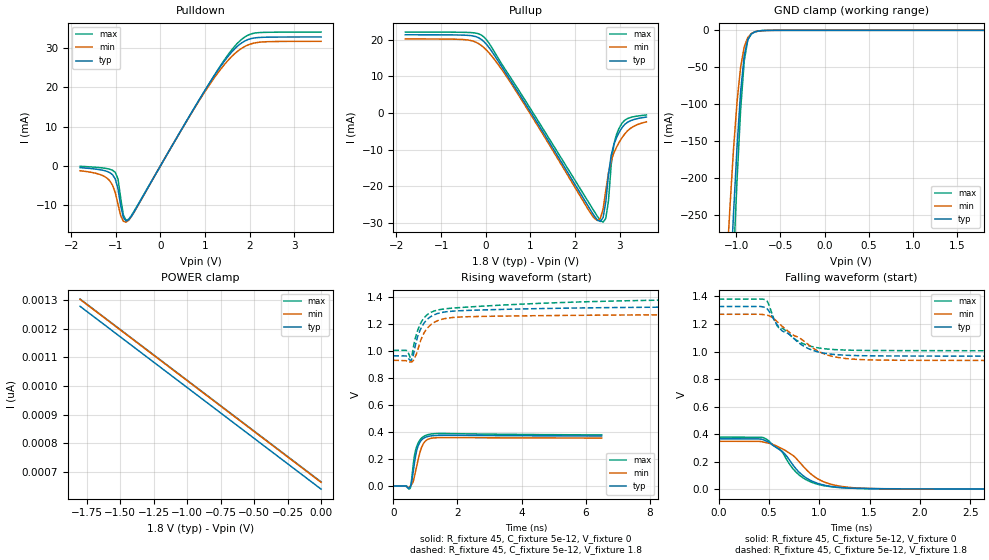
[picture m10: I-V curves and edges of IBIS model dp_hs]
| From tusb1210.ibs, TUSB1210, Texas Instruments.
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|   Model: dp_hs
|   Description:  DP in high-Speed mode
[Model]   dp_hs
Model_type   I/O
Polarity   Non-Inverting
Enable   Active-High
Vmeas =   0.300
Vref =   0
Cref =   5e-12
Rref =   45
|variable   typ   min   max
C_comp   8.0p   7.14p   8.83p
[Receiver Thresholds]
Vcross_low =   -50m
Vcross_high =   500m
Vdiff_ac =   150m
Vdiff_dc =   100m
Tdiffslew_ac =   600p
[Temperature Range]   27   125   -40
[Voltage Range]   1.8   1.728   1.872
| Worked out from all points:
|   slope of the pulldown table from 0 to 0.27 V, typ, clamps not added: 50.6 ohm
|   slope of the pullup table from 0 to 0.27 V, typ, clamps not added: 58.4 ohm
|   GND clamp passes 1 mA (typ) near -0.75 V on its own axis
|   rising waveform, R_fixture 45, C_fixture 5e-12, V_fixture 0: 20-80 % time 172ps typ, 220ps min, 162ps max; typ from 0.001 V to 0.37 V
|   rising waveform, R_fixture 45, C_fixture 5e-12, V_fixture 1.8: 20-80 % time 499ps typ, 478ps min, 816ps max; typ from 0.962 V to 1.33 V
|   falling waveform, R_fixture 45, C_fixture 5e-12, V_fixture 0: 20-80 % time 296ps typ, 330ps min, 272ps max; typ from 0.367 V to 0.001 V
|   falling waveform, R_fixture 45, C_fixture 5e-12, V_fixture 1.8: 20-80 % time 322ps typ, 398ps min, 267ps max; typ from 1.33 V to 0.962 V
[GND Clamp]
| dp_hs
|Voltage   I(typ)   I(min)   I(max)
-1.8V     -2.571A    -2.176A    -2.872A
-1.112V   -460.6mA   -327.5mA   -556.3mA
-1.072V   -351.4mA   -239.8mA   -431.6mA
-1.032V   -248.8mA   -161.3mA   -312.3mA
-991mV    -156.9mA   -96.29mA   -201.7mA
-950.6mV  -82.5mA    -49.52mA   -107mA
-910.1mV  -34.34mA   -22.33mA   -41.35mA
-869.7mV  -12.47mA   -9.64mA    -12.7mA
-829.2mV  -4.861mA   -4.33mA    -4.529mA
-748.3mV  -947.7uA   -1.01mA    -769.6uA
-627mV    -70.16uA   -118.5uA   -34.18uA
1.8V      639.2pA    688.7pA    639pA
[POWER Clamp]
| dp_hs
|Voltage   I(typ)   I(min)   I(max)
-1.8V     1.278nA    1.302nA    1.304nA
-1.699V   1.242nA    1.266nA    1.268nA
-1.557V   1.192nA    1.216nA    1.217nA
0V        639.2pA    663.1pA    664.5pA
[Pulldown]
| dp_hs
|Voltage   I(typ)   I(min)   I(max)
-1.8V     -490.6uA   -1.273mA   -138.8uA
-1.254V   -1.247mA   -2.729mA   -619.8uA
-1.133V   -1.768mA   -3.868mA   -896.7uA
-1.011V   -3.378mA   -6.894mA   -1.704mA
-950.6mV  -5.918mA   -9.83mA    -3.386mA
-829.2mV  -13.22mA   -14.21mA   -12.63mA
-707.9mV  -13.78mA   -13.87mA   -13.65mA
930.3mV   18.02mA    17.75mA    17.96mA
1.355V    25.5mA     24.74mA    25.72mA
1.719V    30.47mA    29.17mA    31.23mA
2.144V    32.71mA    31.45mA    33.95mA
3.6V      32.91mA    31.8mA     34.15mA
[Pullup]
| dp_hs
|Voltage   I(typ)   I(min)   I(max)
-1.8V     21.4mA     20.27mA    22.13mA
-40.4mV   19.53mA    17.89mA    20.8mA
627mV     7.556mA    7.005mA    8.386mA
2.386V    -27.26mA   -28.05mA   -26mA
2.508V    -29.32mA   -29.35mA   -28.34mA
2.629V    -28.56mA   -26.26mA   -29.84mA
2.69V     -24.37mA   -21.23mA   -28.8mA
2.751V    -16.79mA   -16.3mA    -23.96mA
2.811V    -11.48mA   -13.05mA   -14.12mA
2.933V    -6.671mA   -9.267mA   -5.776mA
3.115V    -3.097mA   -5.713mA   -1.953mA
3.6V      -1.095mA   -2.399mA   -525.1uA
[Ramp]
| dp_hs
|variable   typ   min   max
dV/dt_r   0.366/1.686e-10   0.348/2.134e-10   0.378/1.624e-10
dV/dt_f   0.365/3.382e-10   0.341/4.263e-10   0.378/2.778e-10
R_load =   45
[Rising Waveform]
| dp_hs
R_fixture =   45
C_fixture =   5e-12
V_fixture =   0
V_fixture_min =   0
V_fixture_max =   0
|Time   V(typ)   V(min)   V(max)
0s        822.9uV    835.9uV    806.3uV
419.6ps   -5.59mV    -5.875mV   938uV
525.5ps   -4.134mV   -372.3uV   -14.49mV
564.8ps   21.71mV    11.22mV    37.9mV
649.8ps   155mV      62.48mV    211mV
728.9ps   261.9mV    147mV      291.8mV
793.7ps   308.3mV    215mV      327.2mV
889.6ps   342.9mV    290.7mV    356.8mV
1.081ns   367mV      346mV      380.5mV
6.498ns   370.1mV    355mV      378.4mV
[Rising Waveform]
| dp_hs
R_fixture =   45
C_fixture =   5e-12
V_fixture =   1.8
V_fixture_min =   1.728
V_fixture_max =   1.872
|Time   V(typ)   V(min)   V(max)
0s        962.4mV    929.6mV    1.002V
430.6ps   953mV      921mV      1V
554.2ps   928.4mV    917.9mV    951.2mV
616ps     961mV      924.9mV    1.011V
739.6ps   1.089V     987.8mV    1.137V
955.9ps   1.203V     1.13V      1.241V
1.274ns   1.266V     1.21V      1.293V
1.856ns   1.292V     1.245V     1.315V
8.165ns   1.321V     1.265V     1.373V
20.67ns   1.327V     1.271V     1.381V
[Falling Waveform]
| dp_hs
R_fixture =   45
C_fixture =   5e-12
V_fixture =   0
V_fixture_min =   0
V_fixture_max =   0
|Time   V(typ)   V(min)   V(max)
0s        366.6mV    348.5mV    378.4mV
444ps     359.1mV    343.4mV    374.9mV
608.9ps   286.3mV    301.9mV    288.8mV
661.4ps   253.2mV    282.3mV    234.7mV
748.1ps   167.5mV    240.4mV    141.2mV
860.8ps   87.27mV    151mV      73.29mV
1.024ns   34.79mV    60.88mV    29.13mV
1.268ns   10.14mV    16.12mV    9.51mV
1.919ns   2.859mV    2.498mV    3.396mV
9.249ns   824.6uV    849.8uV    806.3uV
[Falling Waveform]
| dp_hs
R_fixture =   45
C_fixture =   5e-12
V_fixture =   1.8
V_fixture_min =   1.728
V_fixture_max =   1.872
|Time   V(typ)   V(min)   V(max)
0s        1.327V     1.271V     1.381V
463.6ps   1.319V     1.266V     1.376V
490.2ps   1.304V     1.262V     1.355V
552.5ps   1.229V     1.236V     1.231V
588.1ps   1.188V     1.213V     1.181V
645.9ps   1.144V     1.174V     1.164V
779.3ps   1.074V     1.107V     1.08V
1.006ns   994.7mV    996.3mV    1.025V
1.255ns   973.6mV    949.8mV    1.011V
13.25ns   962.4mV    929.6mV    1.002V
